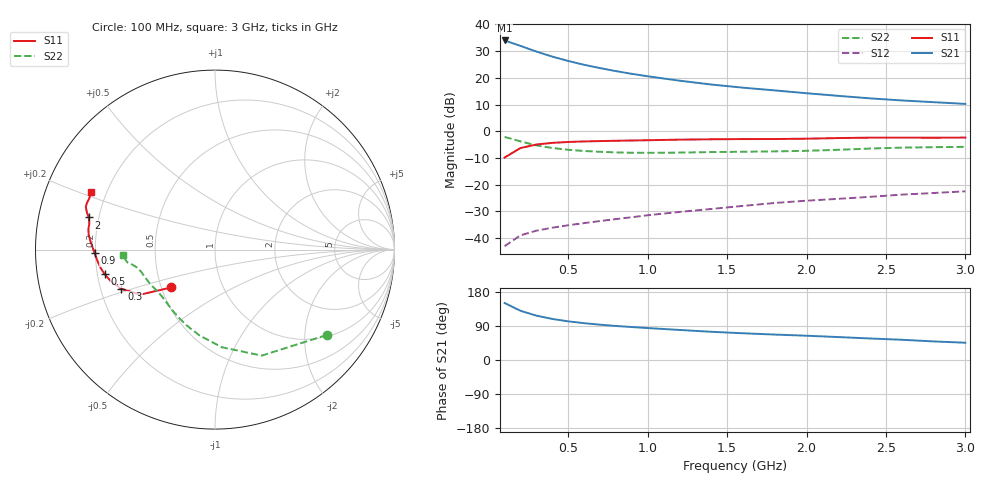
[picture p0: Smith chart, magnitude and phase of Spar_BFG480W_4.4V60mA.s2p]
! Filename: 4_460BFG480.001
! Title: BFG480W
! Bias: Vce=4.4V; Ic=60mA
! Company: NXP Semiconductors NL
! User: Quality&Reliability T&D
! Measure time: 10 Nov 1999 / 12:06:13
#  MHz  S  MA  R 50
! Freq  S11  S21  S12  S22  :
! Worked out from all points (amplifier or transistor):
!   20 points, 100 MHz to 3 GHz, reference 50 ohm
!   highest |S21| = 34.0 dB at 100 MHz (marker M1)
!   |S21| within 3 dB of that: start of sweep to 245.4 MHz
!   unconditionally stable (mu >= 1): 882.9 MHz to end of sweep
!   at 400 MHz: K = 0.70, MSG = 32.0 dB, |S12| = -36.1 dB
!   at 1.2 GHz: K = 1.06, MAG = 23.1 dB, |S12| = -30.2 dB
!   at 3 GHz: K = 1.05, MAG = 15.0 dB, |S12| = -22.5 dB
!   S11 on the Smith chart (normalised r, x): 100 MHz: 0.56, -0.26; 300 MHz: 0.29, -0.19; 500 MHz: 0.23, -0.10; 900 MHz: 0.20, -0.01; 2 GHz: 0.16, +0.12; 3 GHz: 0.14, +0.22
100  0.3216 -139.1  50.2 150.3  0.007047 65.6  0.7839 -37.4
200  0.4857 -148.9  39.71 129.9  0.01126 57.0  0.6455 -66.2
300  0.5652 -157.2  31.09 117.0  0.01375 54.3  0.5452 -86.1
400  0.606 -163.0  25 108.3  0.01562 54.7  0.4856 -100.3
500  0.6299 -167.4  20.74 102.0  0.01736 56.2  0.4499 -110.9
600  0.6449 -170.8  17.59 97.1  0.01903 57.7  0.4275 -119.0
700  0.655 -173.7  15.24 93.2  0.02081 60.0  0.4124 -125.3
800  0.6634 -176.2  13.39 89.9  0.02265 62.2  0.4024 -130.6
900  0.6715 -178.5  11.91 87.0  0.02455 64.3  0.3964 -135.2
1000  0.6798 179.5  10.72 84.3  0.02671 65.8  0.3943 -139.4
1200  0.6962 176.0  8.861 79.3  0.03084 68.3  0.3987 -146.1
1400  0.7081 173.4  7.51 74.5  0.03506 70.0  0.4076 -151.2
1600  0.7143 170.9  6.553 70.6  0.04002 71.5  0.4135 -155.1
1800  0.7154 168.2  5.825 67.1  0.04538 72.6  0.4201 -159.0
2000  0.726 165.7  5.157 64.1  0.05008 73.7  0.4303 -163.6
2200  0.746 163.5  4.605 60.5  0.05429 74.0  0.4496 -167.6
2400  0.7585 161.6  4.132 56.8  0.05912 73.8  0.4743 -170.3
2600  0.7593 160.0  3.777 53.4  0.06506 73.4  0.4938 -171.8
2800  0.7564 157.7  3.506 49.0  0.06981 72.3  0.5032 -173.8
3000  0.7615 155.0  3.256 45.6  0.07509 71.7  0.5107 -176.8
